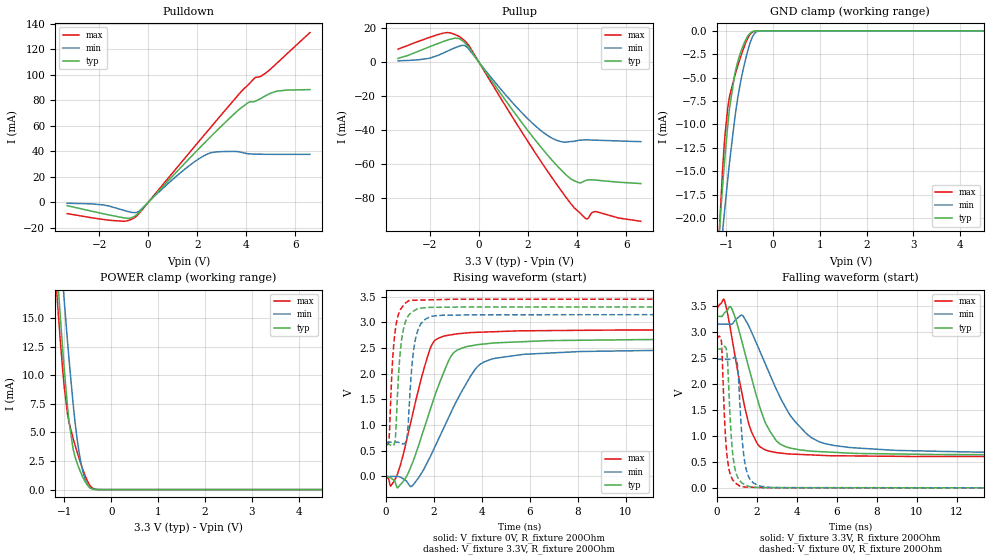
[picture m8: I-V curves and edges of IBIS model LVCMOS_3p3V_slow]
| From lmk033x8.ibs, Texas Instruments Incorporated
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[Model]   LVCMOS_3p3V_slow
Model_type   3-state
Polarity   Non-Inverting
Vmeas = 1.65
Vref = 3.3
Cref = 15pF
Rref = 200
|   typ   min   max
|   (nom PVT)   (fast PVT)   (slow PVT)
C_comp   0.571p   0.551p   0.636p
|C_comp (ON state)   0.658p   0.615p   0.711p
|C_comp (OFF state)   0.571p   0.551p   0.636p
[Voltage Range]   3.3   3.15   3.45
[Temperature Range]   27   125   -40
[Pullup Reference]   3.3   3.15   3.45
[Pulldown Reference]   -0   -0   0
[Power Clamp Reference]   3.3   3.15   3.45
[GND Clamp Reference]   0   0   0
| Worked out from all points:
|   slope of the pulldown table from 0 to 0.495 V, typ, clamps not added: 48 ohm
|   slope of the pullup table from 0 to 0.495 V, typ, clamps not added: 47.7 ohm
|   GND clamp passes 1 mA (typ) near -0.58 V on its own axis
|   POWER clamp passes 1 mA (typ) near -0.60 V on its own axis
|   falling waveform, V_fixture 3.3V, R_fixture 200Ohm: 20-80 % time 1.26ns typ, 2.05ns min, 890ps max; typ from 3.3 V to 0.632 V
|   rising waveform, V_fixture 0V, R_fixture 200Ohm: 20-80 % time 1.2ns typ, 1.6ns min, 910ps max; typ from 0.001 V to 2.67 V
|   rising waveform, V_fixture 3.3V, R_fixture 200Ohm: 20-80 % time 248ps typ, 278ps min, 227ps max; typ from 0.63 V to 3.3 V
|   falling waveform, V_fixture 0V, R_fixture 200Ohm: 20-80 % time 261ps typ, 296ps min, 233ps max; typ from 2.67 V to 0 V
[Pulldown]
|   Voltage   I(typ)   I(min)   I(max)
-3.3V     -2.52mA    -600.3uA   -8.758mA
-1.865V   -8.706mA   -1.855mA   -13.25mA
-963.6mV  -12.15mA   -6.33mA    -14.77mA
-528mV    -10.55mA   -7.967mA   -11.61mA
-379.5mV  -7.92mA    -6.939mA   -8.819mA
1.541V    31.66mA    26.77mA    35.73mA
2.511V    50.79mA    38.65mA    57.96mA
3.482V    68.92mA    40.03mA    79.92mA
4.125V    78.74mA    38.11mA    93.15mA
4.372V    79.36mA    37.88mA    97.98mA
5.273V    87.34mA    37.74mA    109.6mA
6.6V      88.5mA     37.75mA    133.2mA
[GND Clamp]
|   Voltage   I(typ)   I(min)   I(max)
-3.3V     -203.8mA   -156.3mA   -307mA
-1.171V   -23.41mA   -26.67mA   -23.99mA
-1.073V   -16.48mA   -21.32mA   -14.64mA
-1.053V   -15.2mA    -20.29mA   -13.1mA
-1.023V   -13.35mA   -18.76mA   -11.08mA
-963.6mV  -10.02mA   -15.81mA   -8.174mA
-924mV    -8.154mA   -13.94mA   -6.971mA
-815.1mV  -4.636mA   -9.357mA   -4.815mA
-636.9mV  -1.582mA   -4.164mA   -2.006mA
-438.9mV  -95.08uA   -660.3uA   -145.6uA
-260.7mV  -658.8nA   -9.216uA   -902.5nA
6.6V      0A         0A         0A
[Pullup]
|   Voltage   I(typ)   I(min)   I(max)
-3.3V     2.259mA    815.6uA    7.66mA
-2.072V   8.734mA    2.189mA    14.32mA
-1.439V   12.24mA    5.483mA    17.14mA
-815.1mV  13.98mA    9.403mA    15.2mA
-468.6mV  9.775mA    8.571mA    10.86mA
1.264V    -26.02mA   -22.09mA   -29.92mA
2.511V    -49.62mA   -40mA      -57.94mA
3.204V    -61.15mA   -46.09mA   -72.5mA
3.897V    -69.75mA   -46.44mA   -85.74mA
4.402V    -69.29mA   -45.69mA   -92.17mA
4.749V    -69.29mA   -45.82mA   -87.72mA
6.6V      -71.34mA   -46.7mA    -93.52mA
[POWER Clamp]
|   Voltage   I(typ)   I(min)   I(max)
-3.3V     163.1mA    154.7mA    175.2mA
-1.162V   19.42mA    25.01mA    17.09mA
-1.092V   15.36mA    21.2mA     13.24mA
-1.013V   11.02mA    16.97mA    9.368mA
-933.9mV  7.229mA    12.94mA    6.584mA
-904.2mV  6.039mA    11.5mA     5.927mA
-815.1mV  3.558mA    7.522mA    4.491mA
-716.1mV  2.165mA    4.038mA    3.108mA
-656.7mV  1.543mA    2.548mA    2.342mA
-567.6mV  770.8uA    1.019mA    1.318mA
-409.2mV  60.75uA    64.51uA    154.9uA
6.6V      0A         0A         0A
[Ramp]
R_load = 200
|   typ   min   max
dV/dt_r   1.60181/1.19368e-09   1.48097/1.60249e-09   1.71223/9.06296e-10
dV/dt_f   1.60083/1.25683e-09   1.48593/2.04325e-09   1.70887/8.89594e-10
[Falling Waveform]
V_fixture = 3.3V
V_fixture_min = 3.15V
V_fixture_max = 3.45V
R_fixture = 200Ohm
C_fixture = 0F
|   Time   V(typ)   V(min)   V(max)
0s        3.3V       3.15V      3.447V
354.8ps   3.35V      3.149V     3.63V
762.7ps   3.437V     3.152V     2.88V
1.251ns   2.828V     3.326V     1.84V
1.618ns   2.291V     3.101V     1.213V
2.408ns   1.277V     2.406V     733.5mV
3.008ns   896mV      1.876V     677.6mV
3.729ns   761.8mV    1.368V     650.4mV
5.385ns   693mV      855.1mV    623mV
19ns      632mV      673.5mV    599.2mV
[Rising Waveform]
V_fixture = 0V
V_fixture_min = 0V
V_fixture_max = 0V
R_fixture = 200Ohm
C_fixture = 0F
|   Time   V(typ)   V(min)   V(max)
0s        1.235mV    65.83nV    -137.8nV
344.8ps   -78.75mV   1.524mV    -91.48mV
852.6ps   -6.246mV   -88.28mV   682.7mV
1.132ns   294mV      -165.2mV   1.245V
1.819ns   1.257V     355.8mV    2.45V
2.352ns   1.954V     883.7mV    2.719V
2.961ns   2.455V     1.479V     2.774V
3.774ns   2.56V      2.114V     2.804V
4.561ns   2.599V     2.3V       2.817V
19ns      2.671V     2.468V     2.854V
[Rising Waveform]
V_fixture = 3.3V
V_fixture_min = 3.15V
V_fixture_max = 3.45V
R_fixture = 200Ohm
C_fixture = 0F
|   Time   V(typ)   V(min)   V(max)
0s        630.5mV    665mV      610mV
130.8ps   622.5mV    666.3mV    718.7mV
274.8ps   596.7mV    667.8mV    2.229V
420.5ps   941.8mV    669.3mV    2.941V
615.6ps   2.502V     648.7mV    3.255V
849.5ps   3.052V     699mV      3.386V
965.8ps   3.147V     1.314V     3.423V
1.242ns   3.243V     2.693V     3.43V
1.938ns   3.29V      3.119V     3.437V
19ns      3.3V       3.15V      3.45V
[Falling Waveform]
|Gnd
V_fixture = 0V
V_fixture_min = 0V
V_fixture_max = 0V
R_fixture = 200Ohm
C_fixture = 0F
|   Time   V(typ)   V(min)   V(max)
0s        2.674V     2.474V     2.863V
235.5ps   2.672V     2.473V     2.809V
420.5ps   2.715V     2.473V     1.099V
586.6ps   2.057V     2.472V     410.3mV
808.5ps   622.8mV    2.493V     147.4mV
1.027ns   223.4mV    2.394V     68.01mV
1.192ns   122.7mV    1.386V     22.68mV
1.533ns   39.37mV    273.2mV    15.06mV
2.241ns   6.824mV    28.57mV    4.594mV
19ns      107.4uV    167.6uV    71.6uV
